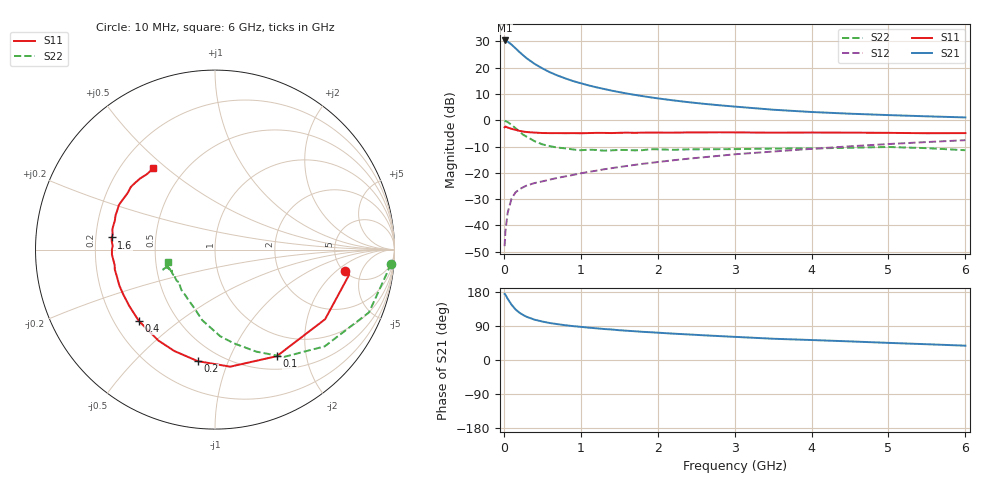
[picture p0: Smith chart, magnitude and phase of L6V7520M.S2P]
!  INFINEON TECHNOLOGIES Small Signal Semiconductors
! BFR380L3 , Si-NPN RF-Transistor in TSLP-3-1
!  Vce=0.75 V,  Ic=20 mA
! Common Emitter S-Parameters:  07. March 2005
#  GHz  S  MA  R  50
! f  S11  S21  S12  S22
! GHz  Mag  Ang  Mag  Ang  Mag  Ang  Mag  Ang
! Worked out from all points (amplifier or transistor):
!   36 points, 10 MHz to 6 GHz, reference 50 ohm
!   highest |S21| = 30.4 dB at 10 MHz (marker M1)
!   |S21| within 3 dB of that: start of sweep to 152.7 MHz
!   unconditionally stable (mu >= 1): 1.66 GHz to 5.543 GHz
!   at 250 MHz: K = 0.38, MSG = 25.2 dB, |S12| = -25.5 dB
!   at 1.4 GHz: K = 0.97, MSG = 14.8 dB, |S12| = -18.3 dB
!   at 6 GHz: K = 0.99, MSG = 4.3 dB, |S12| = -7.6 dB
!   S11 on the Smith chart (normalised r, x): 10 MHz: 5.16, -2.64; 100 MHz: 0.68, -1.52; 200 MHz: 0.38, -0.78; 400 MHz: 0.30, -0.36; 1.6 GHz: 0.27, +0.05; 6 GHz: 0.34, +0.45
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0.01  0.7351 -9.2  33.09 174.4  0.004 82.5  0.9842 -4.6
0.02  0.7605 -10.6  32.93 172.6  0.0075 87.2  0.96 -9.2
0.05  0.7259 -32.3  31.43 161.4  0.0174 77.0  0.9266 -22.2
0.1  0.6863 -59.9  27.59 145.9  0.0322 65.0  0.815 -41.4
0.15  0.6578 -82.6  23.63 133.9  0.042 56.4  0.7106 -57.3
0.2  0.6288 -98.8  20.1 125.2  0.0483 52.3  0.613 -68.0
0.25  0.6089 -111.8  17.34 118.9  0.0529 48.8  0.532 -78.7
0.3  0.5968 -121.9  15.02 113.7  0.0575 47.3  0.4833 -86.6
0.4  0.5815 -136.8  11.86 106.4  0.0637 46.7  0.3991 -100.4
0.5  0.5717 -146.8  9.739 101.5  0.0685 47.5  0.3479 -108.9
0.6  0.5688 -154.0  8.182 97.5  0.0742 48.8  0.3205 -116.8
0.7  0.5693 -159.3  7.104 94.5  0.0801 50.6  0.3013 -124.0
0.9  0.5691 -168.8  5.575 89.4  0.091 53.0  0.2777 -135.1
1.1  0.57 -174.6  4.618 85.4  0.1039 55.5  0.275 -140.4
1.3  0.5742 179.8  3.949 81.8  0.1163 57.2  0.2635 -147.6
1.6  0.5805 173.3  3.229 77.2  0.1348 58.6  0.2716 -153.3
2.2  0.5811 163.7  2.394 69.6  0.173 60.3  0.2734 -156.0
2.8  0.5904 155.2  1.93 63.1  0.2106 61.0  0.2815 -160.5
3.5  0.5799 146.8  1.588 56.1  0.2536 59.4  0.2886 -159.9
4.5  0.5806 140.4  1.333 49.1  0.3192 57.9  0.2997 -159.6
5.5  0.5661 132.1  1.188 41.6  0.3847 53.9  0.2943 -160.6
6  0.5694 127.0  1.132 37.8  0.4174 51.7  0.2687 -165.0
